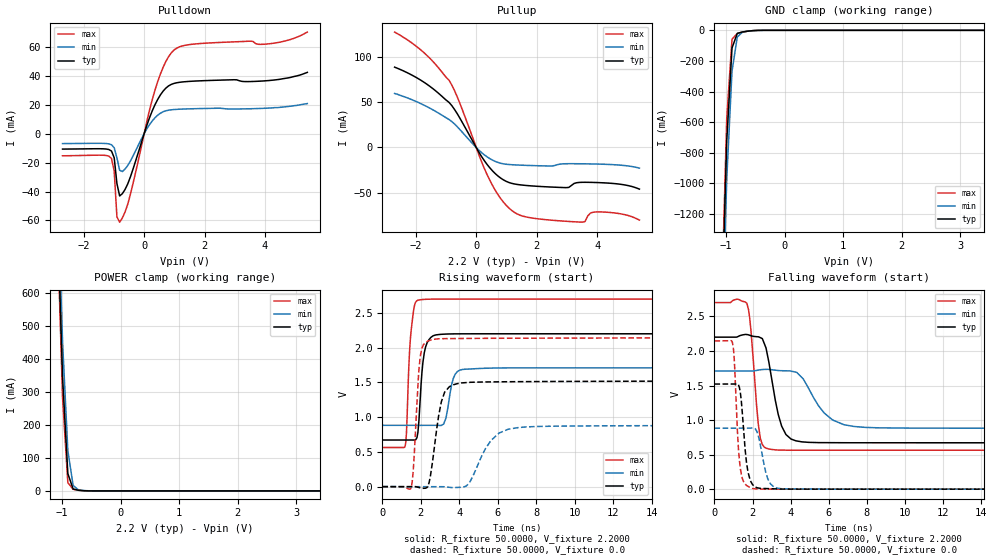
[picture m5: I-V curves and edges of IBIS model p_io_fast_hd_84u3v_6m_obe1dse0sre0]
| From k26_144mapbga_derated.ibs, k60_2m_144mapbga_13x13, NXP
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[Model] p_io_fast_hd_84u3v_6m_obe1dse0sre0
|   Model p_io_fast_hd_84u3v_6m_obe1dse0sre0
| Library cells for typ/min/max conditions are connected as defined below:
|  pad - External Pad
|  ipp_do - Core Input
|  ipp_obe - Output Buffer Enable
|  esd_boost - vdd_s_3v
|  esd_bus - vdd_s_3v
|  ipp_ina40a_3v - NC
|  ipp_ina40b_3v - NC
|  ipp_ina_3v - NC
|  ipp_ind - NC
|  ipp_ind_3v - NC
|  vdd_s_3v - vdd_s_3v
|  vdd_s_lv - vdd_s_lv
|  vss_bulk - vss_bulk
|  vss_s_lv - vss_s_lv
| All other pins connected to ground
Model_type I/O
Polarity   Non-Inverting
Enable   Active-High
Vinl =   0.6600V
Vinh =   1.6500V
Vmeas =  1.1000V
Cref =   25.0000pF
Rref =   50.0000
Vref =   0.0V
C_comp   3.2952pF   3.0151pF   3.6465pF
[Temperature Range]   25.0000   0.1250k   -40.0000
[Voltage Range]   2.2000V   1.7100V   2.7000V
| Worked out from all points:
|   slope of the pulldown table from 0 to 0.33 V, typ, clamps not added: 17.6 ohm
|   slope of the pullup table from 0 to 0.33 V, typ, clamps not added: 19 ohm
|   GND clamp passes 1 mA (typ) near -0.49 V on its own axis
|   POWER clamp passes 1 mA (typ) near -0.65 V on its own axis
|   rising waveform, R_fixture 50.0000, V_fixture 2.2000: 20-80 % time 256ps typ, 328ps min, 222ps max; typ from 0.671 V to 2.2 V
|   rising waveform, R_fixture 50.0000, V_fixture 0.0: 20-80 % time 484ps typ, 1.06ns min, 262ps max; typ from 0 V to 1.52 V
|   falling waveform, R_fixture 50.0000, V_fixture 2.2000: 20-80 % time 643ps typ, 1.23ns min, 360ps max; typ from 2.2 V to 0.671 V
|   falling waveform, R_fixture 50.0000, V_fixture 0.0: 20-80 % time 300ps typ, 410ps min, 237ps max; typ from 1.52 V to 0 V
[Pulldown]
|Voltage   I(typ)   I(min)   I(max)
-2.7V     -10.62mA   -6.81mA    -15.27mA
-1.08V    -11.96mA   -7.61mA    -17.07mA
-990mV    -16.62mA   -9.699mA   -25.88mA
-900mV    -34.47mA   -16.66mA   -57.57mA
-810mV    -43.05mA   -25.29mA   -61.23mA
-450mV    -29.63mA   -18.74mA   -41.62mA
360mV     20.13mA    11.08mA    30.28mA
720mV     31.63mA    15.91mA    50.1mA
990mV     34.87mA    16.77mA    57.99mA
1.98V     36.76mA    17.5mA     62.65mA
4.23V     37.06mA    17.9mA     62.54mA
5.4V      42.5mA     20.9mA     70.4mA
[Pullup]
|Voltage   I(typ)   I(min)   I(max)
-2.7V     88.9mA     59.8mA     127.7mA
-1.71V    71.79mA    46.54mA    104.4mA
-900mV    49.91mA    30.94mA    74.46mA
-630mV    37.51mA    23.06mA    56.23mA
360mV     -18.78mA   -10.4mA    -30.02mA
720mV     -31.59mA   -16.58mA   -52.18mA
1.17V     -39.68mA   -19.05mA   -69.56mA
2.7V      -44.11mA   -18.89mA   -81.03mA
3.51V     -38.55mA   -18.06mA   -82.69mA
3.78V     -38.61mA   -18.21mA   -72.59mA
4.05V     -38.88mA   -18.4mA    -71.3mA
5.4V      -46.1mA    -22.85mA   -80.32mA
[GND_clamp]
|Voltage   I(typ)   I(min)   I(max)
-2.7V     -32.14A    -31.92A    -32.34A
-1.08V    -1.91A     -2.124A    -1.805A
-990mV    -722.5mA   -972.4mA   -577.1mA
-900mV    -115.5mA   -266.4mA   -57.9mA
-810mV    -19.93mA   -43.77mA   -19.98mA
-720mV    -10.39mA   -11.37mA   -12.14mA
-450mV    -352.7uA   -666.6uA   -211.4uA
5.4V      0A         0A         0A
[POWER_clamp]
|Voltage   I(typ)   I(min)   I(max)
-2.7V     12.62A     12.52A     12.72A
-1.08V    845.9mA    937.2mA    801mA
-990mV    343.7mA    450.6mA    281.4mA
-900mV    52.67mA    121.9mA    25.14mA
-810mV    5.857mA    16.75mA    4.96mA
-720mV    2.026mA    3.175mA    2.02mA
-450mV    19.37uA    104.4uA    4.146uA
5.4V      0A         0A         0A
[Ramp]
| variable   typ   min   max
dV/dt_r  0.9126/0.4843n   0.5291/1.0618n   1.2870/0.2615n
dV/dt_f  0.9173/0.6427n   0.4965/1.2331n   1.2820/0.3600n
R_load = 50.0000
[Rising Waveform]
R_fixture= 50.0000
V_fixture= 2.2000
V_fixture_min= 1.7100
V_fixture_max= 2.7000
|time   V(typ)   V(min)   V(max)
0s        671.2mV    882.4mV    563.3mV
1.192ns   671.2mV    882.4mV    592.7mV
1.5ns     671.3mV    882.4mV    2.253V
1.902ns   949.9mV    882.4mV    2.687V
2.059ns   1.648V     882.4mV    2.692V
2.252ns   2.015V     882.4mV    2.696V
2.965ns   2.19V      880.8mV    2.7V
3.782ns   2.199V     1.615V     2.7V
4.324ns   2.2V       1.69V      2.7V
50ns      2.2V       1.71V      2.7V
[Rising Waveform]
R_fixture= 50.0000
V_fixture= 0.0
V_fixture_min= 0.0
V_fixture_max= 0.0
|time   V(typ)   V(min)   V(max)
0s        2.987nV    464.6nV    82.07pV
1.482ns   -5.189uV   857.7nV    -26.53mV
1.971ns   -19.43mV   129nV      1.879V
2.381ns   14.58mV    -3.887uV   2.096V
2.656ns   460.2mV    -3.113uV   2.12V
3.238ns   1.359V     -2.79mV    2.131V
4.129ns   1.493V     -8.976mV   2.133V
5.637ns   1.508V     660.8mV    2.135V
7.487ns   1.512V     859.6mV    2.137V
50ns      1.521V     881.9mV    2.145V
[Falling Waveform]
R_fixture= 50.0000
V_fixture= 2.2000
V_fixture_min= 1.7100
V_fixture_max= 2.7000
|time   V(typ)   V(min)   V(max)
0s        2.2V       1.71V      2.7V
1.701ns   2.237V     1.71V      2.691V
1.922ns   2.22V      1.709V     2.285V
2.404ns   2.193V     1.728V     741.2mV
2.941ns   1.7V       1.731V     577mV
3.528ns   912.7mV    1.714V     565.2mV
4.661ns   683.2mV    1.597V     563.7mV
6.207ns   672.2mV    1.001V     563.5mV
7.912ns   671.5mV    894.2mV    563.3mV
50ns      671.2mV    882.4mV    563.3mV
[Falling Waveform]
R_fixture= 50.0000
V_fixture= 0.0
V_fixture_min= 0.0
V_fixture_max= 0.0
|time   V(typ)   V(min)   V(max)
0s        1.521V     881.9mV    2.146V
950.7ps   1.521V     881.9mV    2.114V
1.04ns    1.52V      881.9mV    1.882V
1.245ns   1.512V     881.9mV    638.2mV
1.353ns   1.412V     881.9mV    313.1mV
1.682ns   388.7mV    881.1mV    53.39mV
1.998ns   67.27mV    886.3mV    8.828mV
2.805ns   6.801mV    145.8mV    515.7uV
3.479ns   1.704mV    7.381mV    51.29uV
50ns      9.836nV    471nV      4.373nV
